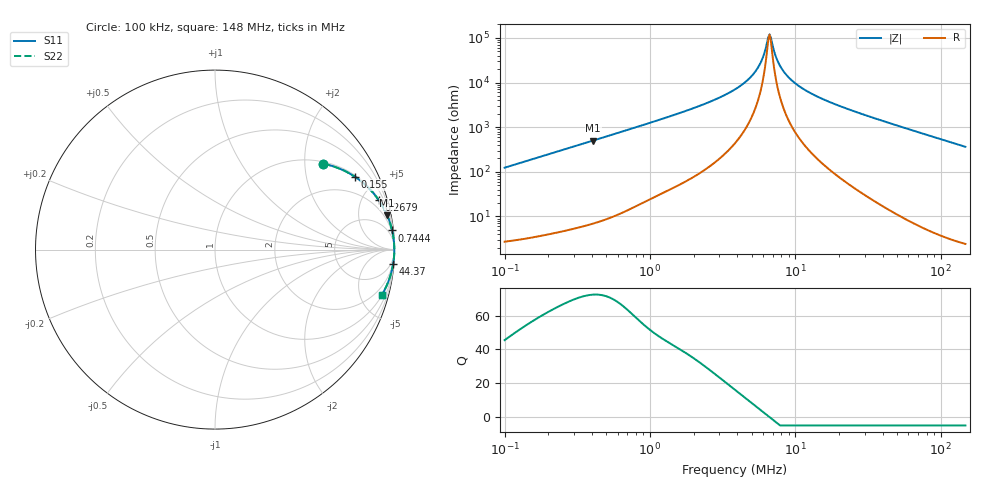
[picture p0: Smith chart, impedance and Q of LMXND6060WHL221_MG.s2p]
! LMXND6060WHL221_MG  S-PARAMETER MODEL  ( Standard Model )
! Model Generated by TAIYO YUDEN Corporation (http://www.ty-top.com)
! Version 1.0
! TAIYO YUDEN Control No. 20240221
! Copyright(c) 2024 TAIYO YUDEN CO.,LTD. All Rights Reserved.
! Product Description (link to TY-COMPAS)
! https://ds.yuden.co.jp/TYCOMPAS/or/detail?pn=LMXND6060WHL221MMG&u=M
! Products Name : Inductors
! Characteristics :
!  Inductance : 220 [uH] , SRF(min) : 2.0 [MHz] , DC Resistance(max) : 1.755 [Ohm]
!  Rated Current : Saturation  400 [mA] , Temp Rise  450 [mA] (40 [degC])
!  Case Size : 6.0 x 6.0 / 0.236 x 0.236 [mm/inch] , Thickness : 2.8 / 0.11 [mm/inch]
!  (Conditions: Temperature = 25 [degC] , DC Bias Current = 0 [A])
! External Node Assignments :
!  1  o---GGG---o  2
! GND o---------o GND
! Frequency Range : 0.1MHz  -  147.97148MHz  [ 402 STEP ]
# MHz S RI R 50
! Freq[MHz].  S11 Real  S11 Imag  S21 Real  S21 Imag  S12 Real  S12 Imag  S22 Real  S22 Imag
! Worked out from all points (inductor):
!   401 points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, 100 kHz to 148 MHz, reference 50 ohm
!   read as one part in series: L = 197 uH near 103.7 kHz
!   highest Q = 72.4 at 407.6 kHz (marker M1), where L = 196 uH
!   self-resonance near 6.53 MHz
!   S11 on the Smith chart (normalised r, x): 100 kHz: 1.05, +2.47; 155 kHz: 1.07, +3.83; 267.9 kHz: 1.10, +6.61; 744.4 kHz: 1, +18; 44.37 MHz: 1, -25; 148 MHz: 1.05, -7.28
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0.1  0.6028 0.4784  0.3972 -0.4784  0.3972 -0.4784  0.6028 0.4784
0.154957  0.7815 0.4045  0.2185 -0.4045  0.2185 -0.4045  0.7815 0.4045
0.267901  0.9127 0.275  0.0873 -0.275  0.0873 -0.275  0.9127 0.275
0.339629  0.9432 0.2245  0.0568 -0.2245  0.0568 -0.2245  0.9432 0.2245
0.407624  0.9595 0.1903  0.0405 -0.1903  0.0405 -0.1903  0.9595 0.1903
0.744387  0.9868 0.1065  0.0132 -0.1065  0.0132 -0.1065  0.9868 0.1065
1.153479  0.9939 0.0682  0.00612 -0.0682  0.00612 -0.0682  0.9939 0.0682
2.482438  0.9982 0.0284  0.00179 -0.0284  0.00179 -0.0284  0.9982 0.0284
3.917549  0.9989 0.0137  0.00107 -0.0137  0.00107 -0.0137  0.9989 0.0137
4.701851  0.9991 0.00871  0.000936 -0.00871  0.000936 -0.00871  0.9991 0.00871
5.440922  0.9991 0.00497  0.000873 -0.00497  0.000873 -0.00497  0.9991 0.00497
5.852942  0.9991 0.00314  0.000853 -0.00314  0.000853 -0.00314  0.9991 0.00314
6.412117  0.9992 0.000882  0.000839 -0.000882  0.000839 -0.000882  0.9992 0.000882
6.65047  0.9992 -1.98e-05  0.000837 1.98e-05  0.000837 1.98e-05  0.9992 -1.98e-05
6.897683  0.9992 -0.000921  0.000836 0.000921  0.000836 0.000921  0.9992 -0.000921
7.55667  0.9992 -0.00318  0.000842 0.00318  0.000842 0.00318  0.9992 -0.00318
8.431079  0.9991 -0.00593  0.000864 0.00593  0.000864 0.00593  0.9991 -0.00593
10.119  0.9991 -0.0107  0.00094 0.0107  0.00094 0.0107  0.9991 -0.0107
13.06453  0.9989 -0.018  0.00115 0.018  0.00115 0.018  0.9989 -0.018
20.99691  0.9979 -0.0351  0.00207 0.0351  0.00207 0.0351  0.9979 -0.0351
44.37094  0.9926 -0.0801  0.00736 0.0801  0.00736 0.0801  0.9926 -0.0801
147.9715  0.9283 -0.2547  0.0717 0.2547  0.0717 0.2547  0.9283 -0.2547
